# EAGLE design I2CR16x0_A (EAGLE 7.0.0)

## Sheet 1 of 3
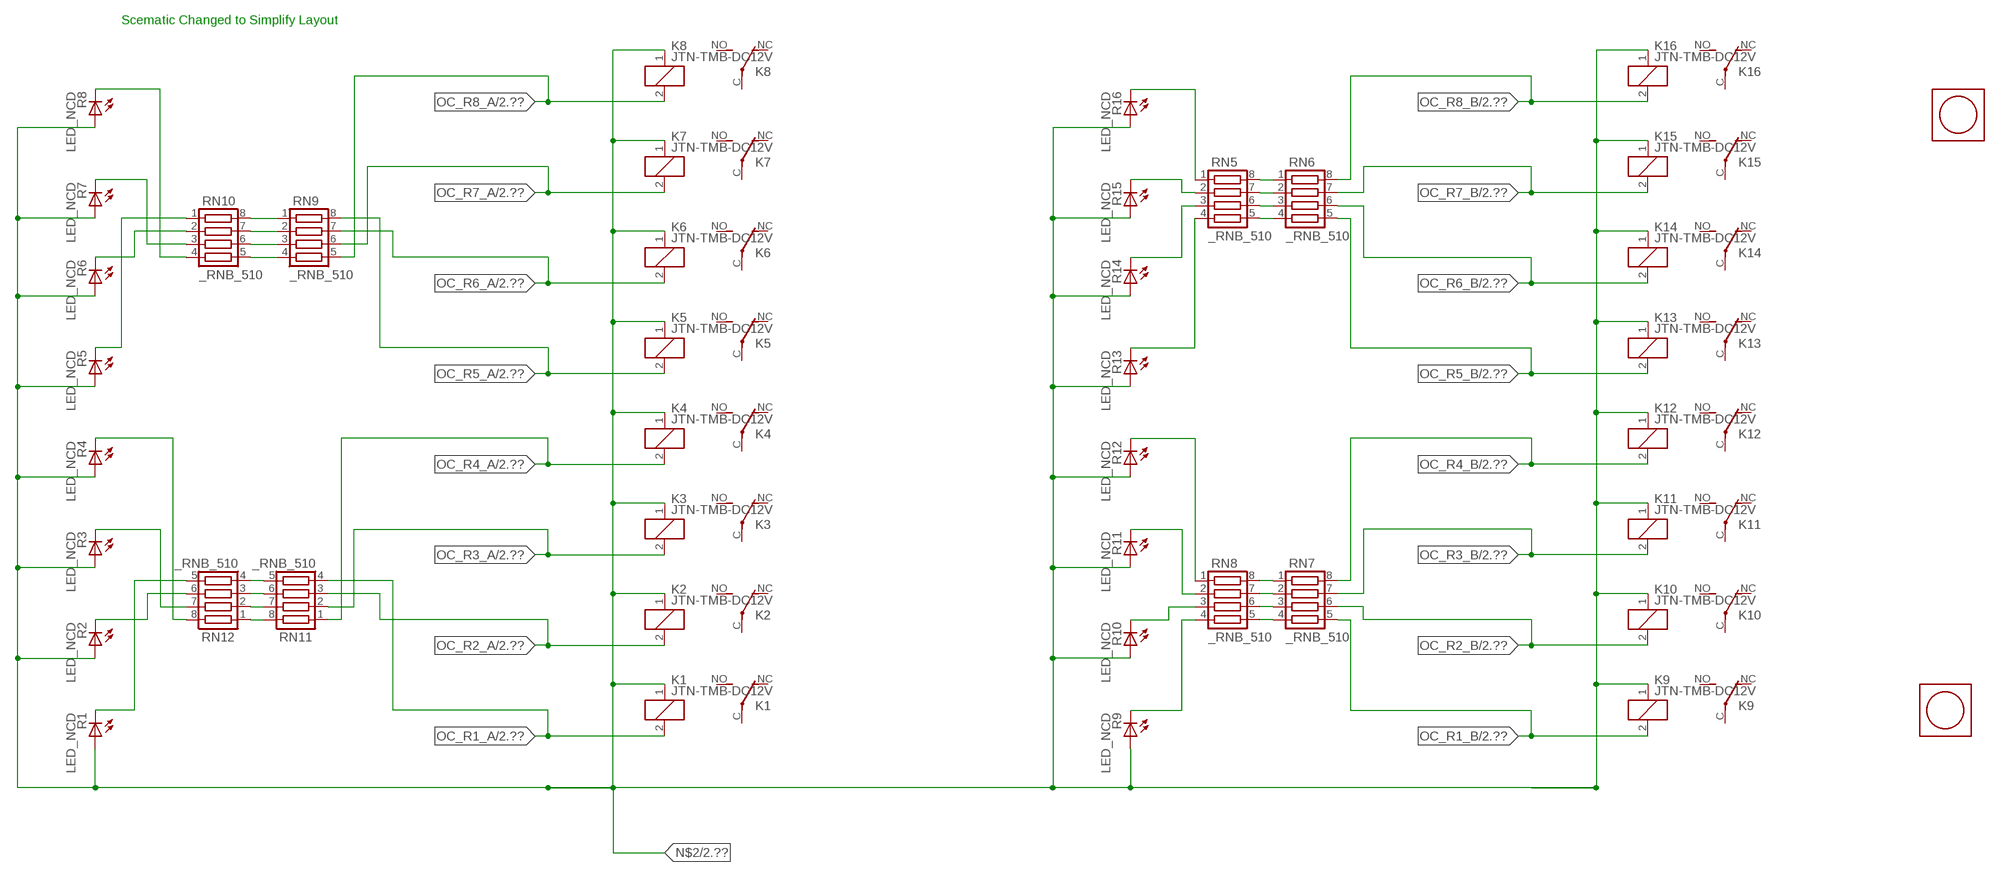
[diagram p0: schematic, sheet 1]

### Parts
K1  JTN-TMB-DC12V  [JT-TMB]
K2  JTN-TMB-DC12V  [JT-TMB]
K3  JTN-TMB-DC12V  [JT-TMB]
K4  JTN-TMB-DC12V  [JT-TMB]
K5  JTN-TMB-DC12V  [JT-TMB]
K6  JTN-TMB-DC12V  [JT-TMB]
K7  JTN-TMB-DC12V  [JT-TMB]
K8  JTN-TMB-DC12V  [JT-TMB]
K9  JTN-TMB-DC12V  [JT-TMB]
K10  JTN-TMB-DC12V  [JT-TMB]
K11  JTN-TMB-DC12V  [JT-TMB]
K12  JTN-TMB-DC12V  [JT-TMB]
K13  JTN-TMB-DC12V  [JT-TMB]
K14  JTN-TMB-DC12V  [JT-TMB]
K15  JTN-TMB-DC12V  [JT-TMB]
K16  JTN-TMB-DC12V  [JT-TMB]
R1  LED_NCD  [CHIPLED_0603]
R2  LED_NCD  [CHIPLED_0603]
R3  LED_NCD  [CHIPLED_0603]
R4  LED_NCD  [CHIPLED_0603]
R5  LED_NCD  [CHIPLED_0603]
R6  LED_NCD  [CHIPLED_0603]
R7  LED_NCD  [CHIPLED_0603]
R8  LED_NCD  [CHIPLED_0603]
R9  LED_NCD  [CHIPLED_0603]
R10  LED_NCD  [CHIPLED_0603]
R11  LED_NCD  [CHIPLED_0603]
R12  LED_NCD  [CHIPLED_0603]
R13  LED_NCD  [CHIPLED_0603]
R14  LED_NCD  [CHIPLED_0603]
R15  LED_NCD  [CHIPLED_0603]
R16  LED_NCD  [CHIPLED_0603]
RN5  _RNB_510  [RNB]
RN6  _RNB_510  [RNB]
RN7  _RNB_510  [RNB]
RN8  _RNB_510  [RNB]
RN9  _RNB_510  [RNB]
RN10  _RNB_510  [RNB]
RN11  _RNB_510  [RNB]
RN12  _RNB_510  [RNB]
U$1  PCB_MOUNTING_HOLE  [PCB_MOUNTING_HOLE]
U$3  PCB_MOUNTING_HOLE  [PCB_MOUNTING_HOLE]

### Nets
N$2: K1.1(C1) K2.1(C1) K3.1(C1) K4.1(C1) K5.1(C1) K6.1(C1) K7.1(C1) K8.1(C1) K9.1(C1) K10.1(C1) K11.1(C1) K12.1(C1) K13.1(C1) K14.1(C1) K15.1(C1) K16.1(C1) R1.A R2.A R3.A R4.A R5.A R6.A R7.A R8.A R9.A R10.A R11.A R12.A R13.A R14.A R15.A R16.A ; also sheet 2,3
N$441: R16.C RN5.1
N$442: RN7.2 RN8.7
N$443: RN7.3 RN8.6
N$444: RN7.4 RN8.5
N$445: R15.C RN5.2
N$447: R13.C RN5.4
N$448: RN5.5 RN6.4
N$449: RN7.1 RN8.8
N$450: R12.C RN8.1
N$451: RN5.6 RN6.3
N$452: R11.C RN8.2
N$453: RN5.7 RN6.2
N$454: RN5.8 RN6.1
N$458: R14.C RN5.3
N$459: R10.C RN8.3
N$463: RN11.5 RN12.4
N$470: R9.C RN8.4
N$473: R1.C RN12.5
N$474: RN11.6 RN12.3
N$475: R2.C RN12.6
N$476: R3.C RN12.7
N$477: RN9.4 RN10.5
N$478: RN9.3 RN10.6
N$479: RN9.2 RN10.7
N$480: RN9.1 RN10.8
N$481: RN11.7 RN12.2
N$482: R5.C RN10.1
N$483: R4.C RN12.8
N$484: R7.C RN10.3
N$485: R8.C RN10.4
N$486: R6.C RN10.2
N$500: RN11.8 RN12.1
OC_R1_A: K1.2(C2) RN11.4 ; also sheet 2
OC_R1_B: K9.2(C2) RN7.5 ; also sheet 2
OC_R2_A: K2.2(C2) RN11.3 ; also sheet 2
OC_R2_B: K10.2(C2) RN7.6 ; also sheet 2
OC_R3_A: K3.2(C2) RN11.2 ; also sheet 2
OC_R3_B: K11.2(C2) RN7.7 ; also sheet 2
OC_R4_A: K4.2(C2) RN11.1 ; also sheet 2
OC_R4_B: K12.2(C2) RN7.8 ; also sheet 2
OC_R5_A: K5.2(C2) RN9.8 ; also sheet 2
OC_R5_B: K13.2(C2) RN6.5 ; also sheet 2
OC_R6_A: K6.2(C2) RN9.7 ; also sheet 2
OC_R6_B: K14.2(C2) RN6.6 ; also sheet 2
OC_R7_A: K7.2(C2) RN9.6 ; also sheet 2
OC_R7_B: K15.2(C2) RN6.7 ; also sheet 2
OC_R8_A: K8.2(C2) RN9.5 ; also sheet 2
OC_R8_B: K16.2(C2) RN6.8 ; also sheet 2
Unconnected: K1.C(COM) K1.NC K1.NO K2.C(COM) K2.NC K2.NO K3.C(COM) K3.NC K3.NO K4.C(COM) K4.NC K4.NO K5.C(COM) K5.NC K5.NO K6.C(COM) K6.NC K6.NO K7.C(COM) K7.NC K7.NO K8.C(COM) K8.NC K8.NO K9.C(COM) K9.NC K9.NO K10.C(COM) K10.NC K10.NO K11.C(COM) K11.NC K11.NO K12.C(COM) K12.NC K12.NO K13.C(COM) K13.NC K13.NO K14.C(COM) K14.NC K14.NO K15.C(COM) K15.NC K15.NO K16.C(COM) K16.NC K16.NO

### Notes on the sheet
- Scematic Changed to Simplify Layout

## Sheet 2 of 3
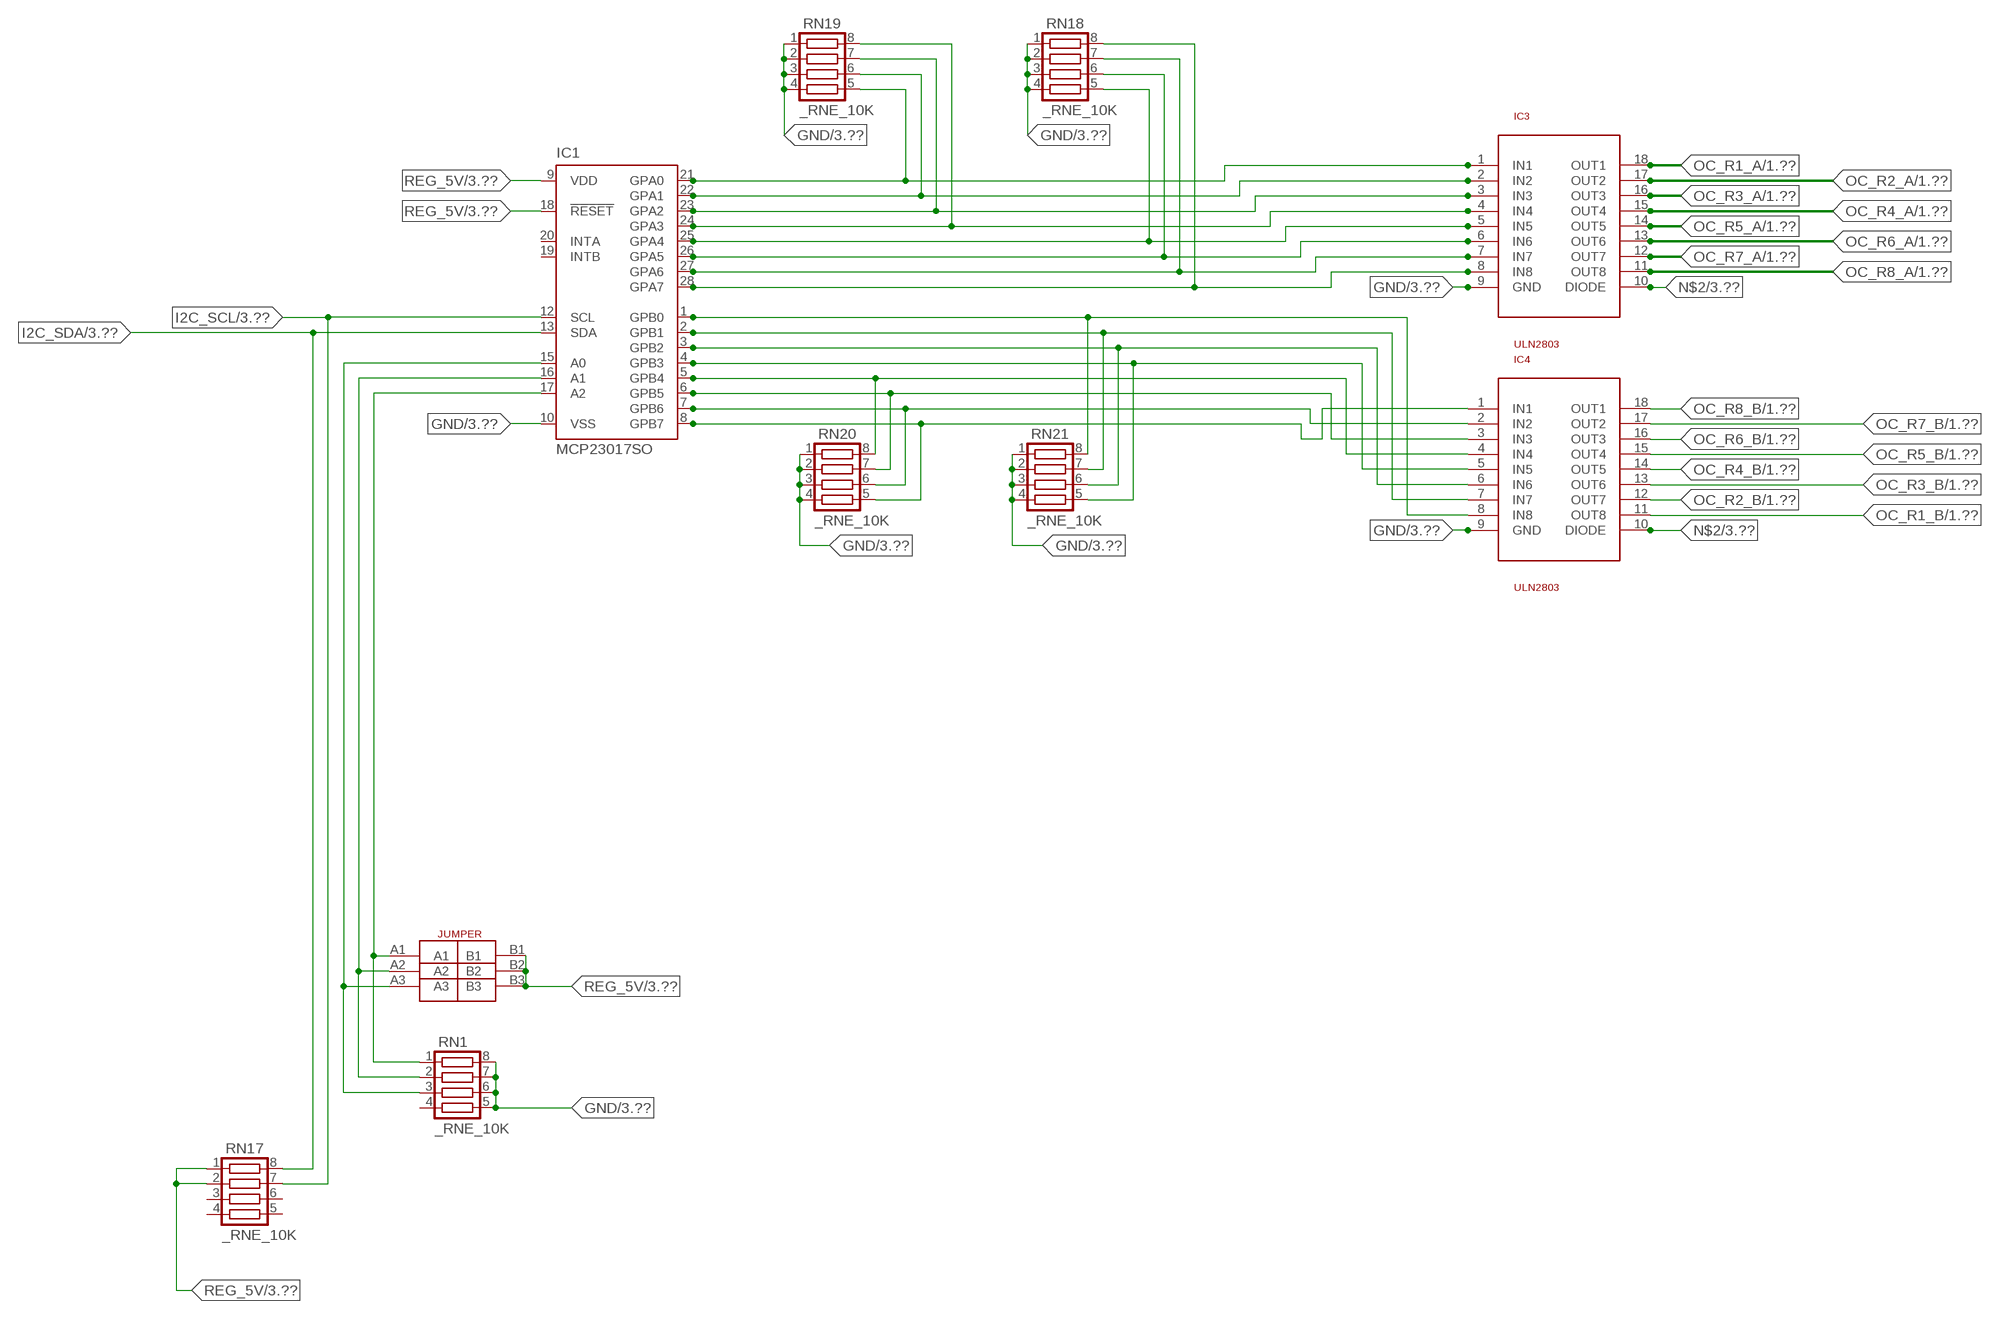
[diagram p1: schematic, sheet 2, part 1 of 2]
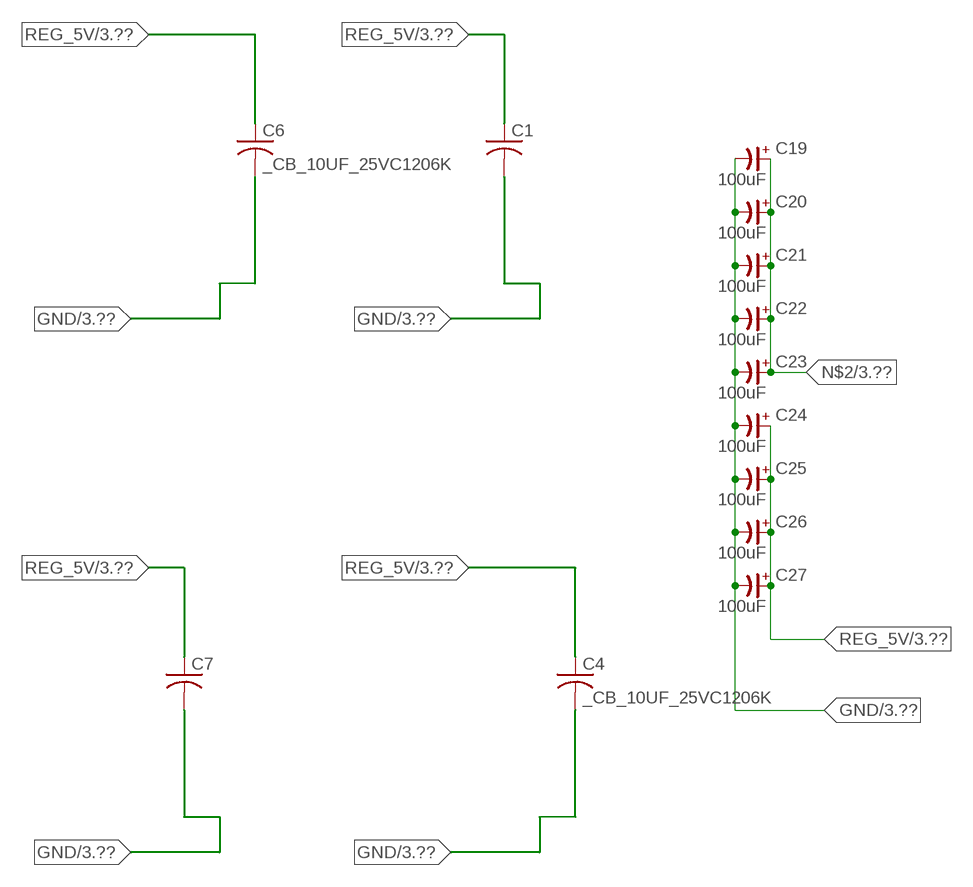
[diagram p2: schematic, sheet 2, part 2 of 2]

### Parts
C1  _CA_.10UF_50VC1206K  [_CA_.1UF_50V]
C4  _CB_10UF_25VC1206K  [_CB_10UF_25V]
C6  _CB_10UF_25VC1206K  [_CB_10UF_25V]
C7  _CA_.10UF_50VC1206K  [_CA_.1UF_50V]
C19  100uF  CP-E-025X060  [E-025X060]
C20  100uF  CP-E-025X060  [E-025X060]
C21  100uF  CP-E-025X060  [E-025X060]
C22  100uF  CP-E-025X060  [E-025X060]
C23  100uF  CP-E-025X060  [E-025X060]
C24  100uF  CP-E-025X060  [E-025X060]
C25  100uF  CP-E-025X060  [E-025X060]
C26  100uF  CP-E-025X060  [E-025X060]
C27  100uF  CP-E-025X060  [E-025X060]
IC1  MCP23017SO  [SO28W]
IC3  ULN2803  [SO18L]
IC4  ULN2803  [SO18L]
JP1  JUMPER_3X2  [JUMPER_3X2]
RN1  _RNE_10K  [RNE]
RN17  _RNE_10K  [RNE]
RN18  _RNE_10K  [RNE]
RN19  _RNE_10K  [RNE]
RN20  _RNE_10K  [RNE]
RN21  _RNE_10K  [RNE]

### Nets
GND: C1.2 C4.2 C6.2 C7.2 C19.- C20.- C21.- C22.- C23.- C24.- C25.- C26.- C27.- IC1.10(VSS) IC3.9(GND) IC4.9(GND) RN1.5 RN1.6 RN1.7 RN1.8 RN18.1 RN18.2 RN18.3 RN18.4 RN19.1 RN19.2 RN19.3 RN19.4 RN20.1 RN20.2 RN20.3 RN20.4 RN21.1 RN21.2 RN21.3 RN21.4 ; also sheet 3
I2C_SCL: IC1.12(SCL) RN17.7 ; also sheet 3
I2C_SDA: IC1.13(SDA) RN17.8 ; also sheet 3
N$2: C19.+ C20.+ C21.+ C22.+ C23.+ IC3.10(DIODE) IC4.10(DIODE) ; also sheet 1,3
N$4: IC1.15(A0) JP1.A3 RN1.3
N$405: IC1.21(GPA0) IC3.1(IN1) RN19.5
N$406: IC1.25(GPA4) IC3.5(IN5) RN18.5
N$407: IC1.26(GPA5) IC3.6(IN6) RN18.6
N$408: IC1.16(A1) JP1.A2 RN1.2
N$409: IC1.22(GPA1) IC3.2(IN2) RN19.6
N$410: IC1.23(GPA2) IC3.3(IN3) RN19.7
N$411: IC1.24(GPA3) IC3.4(IN4) RN19.8
N$416: IC1.1(GPB0) IC4.8(IN8) RN21.8
N$417: IC1.2(GPB1) IC4.7(IN7) RN21.7
N$418: IC1.3(GPB2) IC4.6(IN6) RN21.6
N$419: IC1.4(GPB3) IC4.5(IN5) RN21.5
N$420: IC1.5(GPB4) IC4.4(IN4) RN20.8
N$421: IC1.6(GPB5) IC4.3(IN3) RN20.7
N$422: IC1.7(GPB6) IC4.2(IN2) RN20.6
N$423: IC1.8(GPB7) IC4.1(IN1) RN20.5
N$498: IC1.17(A2) JP1.A1 RN1.1
N$525: IC1.27(GPA6) IC3.7(IN7) RN18.7
N$526: IC1.28(GPA7) IC3.8(IN8) RN18.8
OC_R1_A: IC3.18(OUT1) ; also sheet 1
OC_R1_B: IC4.11(OUT8) ; also sheet 1
OC_R2_A: IC3.17(OUT2) ; also sheet 1
OC_R2_B: IC4.12(OUT7) ; also sheet 1
OC_R3_A: IC3.16(OUT3) ; also sheet 1
OC_R3_B: IC4.13(OUT6) ; also sheet 1
OC_R4_A: IC3.15(OUT4) ; also sheet 1
OC_R4_B: IC4.14(OUT5) ; also sheet 1
OC_R5_A: IC3.14(OUT5) ; also sheet 1
OC_R5_B: IC4.15(OUT4) ; also sheet 1
OC_R6_A: IC3.13(OUT6) ; also sheet 1
OC_R6_B: IC4.16(OUT3) ; also sheet 1
OC_R7_A: IC3.12(OUT7) ; also sheet 1
OC_R7_B: IC4.17(OUT2) ; also sheet 1
OC_R8_A: IC3.11(OUT8) ; also sheet 1
OC_R8_B: IC4.18(OUT1) ; also sheet 1
REG_5V: C1.1 C4.1 C6.1 C7.1 C24.+ C25.+ C26.+ C27.+ IC1.9(VDD) IC1.18(!RESET) JP1.B1 JP1.B2 JP1.B3 RN17.1 RN17.2 ; also sheet 3
Unconnected: IC1.19(INTB) IC1.20(INTA) RN1.4 RN17.3 RN17.4 RN17.5 RN17.6

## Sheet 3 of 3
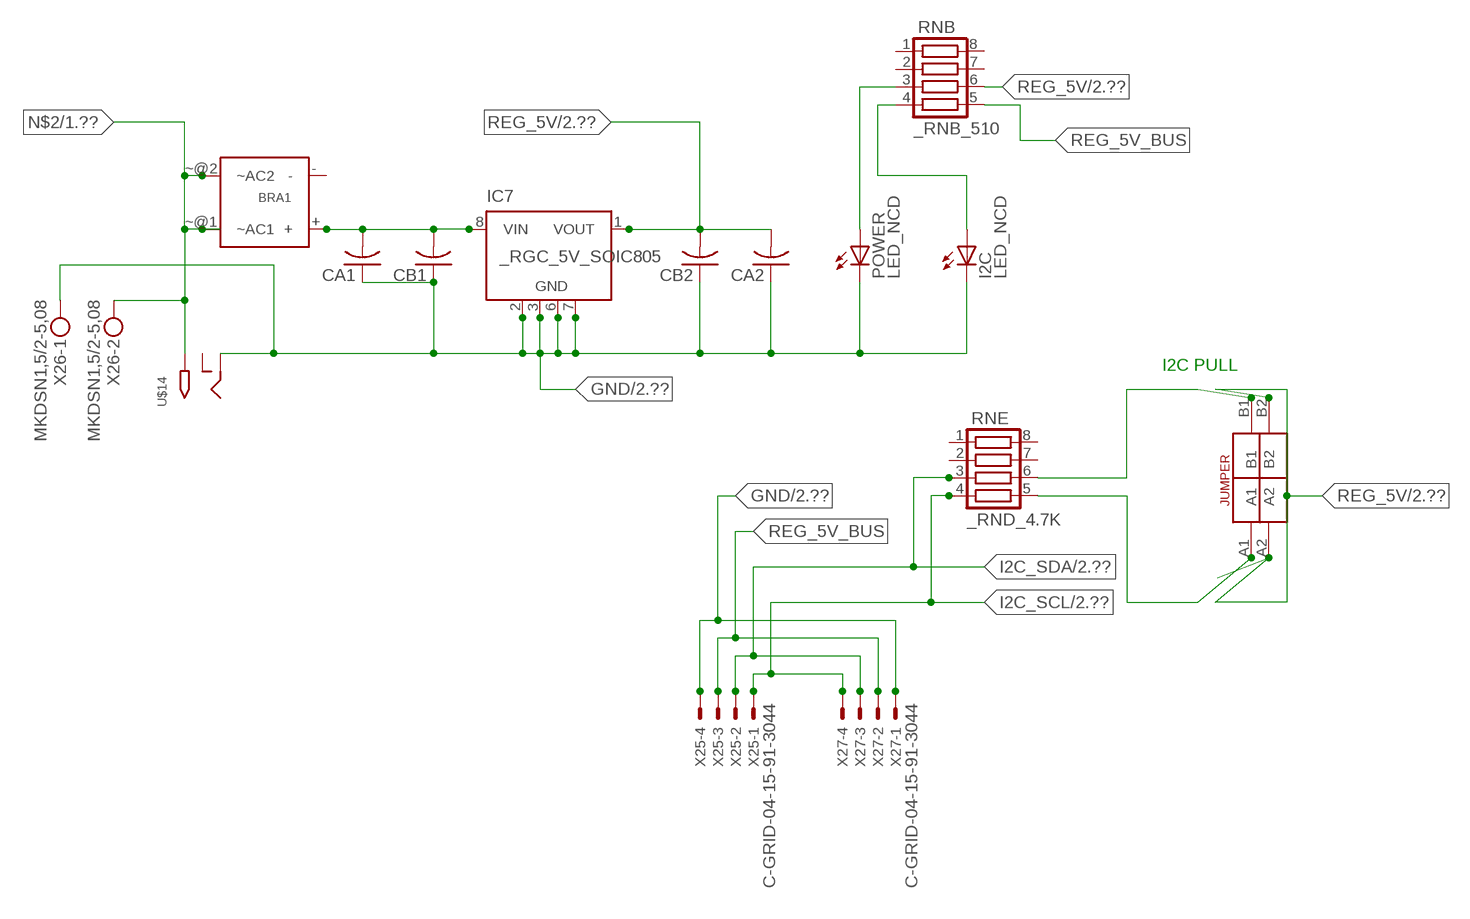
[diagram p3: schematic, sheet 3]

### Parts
BRA1  MB2S_  [MB2S]
CA1  CC1206KRX7R9BB104C1206K  [CC1206KRX7R9BB104]
CA2  CC1206KRX7R9BB104C1206K  [CC1206KRX7R9BB104]
CB1  TMK316F106ZL-TC1206K  [TMK316F106ZL-T]
CB2  TMK316F106ZL-TC1206K  [TMK316F106ZL-T]
I2C  LED_NCD  [CHIPLED_0603]
IC7  _RGC_5V_SOIC805  [_RGC_5V_SOIC8]
POWER  LED_NCD  [CHIPLED_0603]
RNB  _RNB_510  [RNB]
RNE  _RND_4.7K  [RND]
U$14  2.1MMJACK  [PJ-102A]
U$16  JUMPER_2X2  [JUMPER_2X2]
X25  C-GRID-04-15-91-3044  [15-91-04]
X26  MKDSN1,5/2-5,08  [MKDSN1,5/2-5,08]
X27  C-GRID-04-15-91-3044  [15-91-04]

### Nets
GND: CA1.1 CA2.1 CB1.1 CB2.1 I2C.C IC7.2(GND) IC7.3(GND) IC7.6(GND) IC7.7(GND) POWER.C U$14.RING X25.4 X26.1 X27.1 ; also sheet 2
I2C_SCL: RNE.4 X25.1 X27.4 ; also sheet 2
I2C_SDA: RNE.3 X25.2 X27.3 ; also sheet 2
N$2: BRA1.~@1(~AC1) BRA1.~@2(~AC2) U$14.TIP X26.2 ; also sheet 1,2
N$513: BRA1.+ CA1.2 CB1.2 IC7.8(VIN)
N$515: POWER.A RNB.3
N$516: I2C.A RNB.4
N$517: RNE.5 U$16.A1
N$518: RNE.6 U$16.B1
REG_5V: CA2.2 CB2.2 IC7.1(VOUT) RNB.6 U$16.A2 U$16.B2 ; also sheet 2
REG_5V_BUS: RNB.5 X25.3 X27.2
Unconnected: BRA1.- IC7.4(NC) IC7.5(NC) RNB.1 RNB.2 RNB.7 RNB.8 RNE.1 RNE.2 RNE.7 RNE.8 U$14.RING_SW

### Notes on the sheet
- I2C PULL

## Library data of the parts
BRA1 = NCD_ULTIMATE_LIBRARY:MB2S: Bridge Rectifier BRA MB2S 200V 500ma Digikey MB2S-TPMSTR-ND/MB2S-TP
C1 C7 = NCD_ULTIMATE_LIBRARY:_CA_.10UF_50V: Capacitor .1uF SMT
C4 C6 = NCD_ULTIMATE_LIBRARY:_CB_10UF_25V: Capacitor 10uF SMT
C19-C27 = NCD_ULTIMATE_LIBRARY:CP-: Capacitors All Kinds POLARIZED CAP
CA1 CA2 = NCD_ULTIMATE_LIBRARY:CC1206KRX7R9BB104: Capacitor CA .1uF 50V SMT C1206K CC1206KRX7R9BB104
CB1 CB2 = NCD_ULTIMATE_LIBRARY:TMK316F106ZL-T: Capacitor CB 10uF SMT 1206 TMK316F106ZL-T
I2C POWER R1-R16 = NCD_ULTIMATE_bhaskar:LED_NCD
IC1 = NCD_ULTIMATE_LIBRARY:MCP23017: Semiconductor Port Expander I/O 16-Bit I2C http://ww1.microchip.com/downloads/en/DeviceDoc/21952a.pdf Source: http://ww1.microchip.com/downloads/en/DeviceDoc/21952a.pdf
IC3 IC4 = NCD_ULTIMATE_LIBRARY:ULN2803: Semiconductor 8 O.C. N-Channel Transistor Driver Digikey ULN2803AFWGCELTR-ND/ULN2803AFWG,C,EL
IC7 = NCD_ULTIMATE_LIBRARY:_RGC_5V_SOIC8: Regulator Linear 5V Chip Positive VOLTAGE REGULATOR Digikey 497-7267-2-ND/L78L05CD13TR
JP1 = NCD_ULTIMATE_CONNECTORS:JUMPER_3X2
K1-K16 = NCD_ULTIMATE_LIBRARY:JT?-*: RELAY COMPACT ECONOMICAL 30 AMP. RELAY NAiS Source: http://www.mew-europe.com/.. en_ds_61212_0000.pdf
RN1 RN17-RN21 = NCD_ULTIMATE_LIBRARY:_RNE_10K: Resistor Array RNE SMT 10K x 4 Single Resistor Source: http://www.ctscorp.com/components/Datasheets/CTSChipArrayDs.pdf Digikey 742C083103JPTR-ND/742C083103JP; OC_FARNELL: unknown; OC_NEWARK: unknown
RN5-RN12 RNB = NCD_ULTIMATE_LIBRARY:_RNB_510: Resistor Array RNB SMT 510 x 4 Single Resistor Source: http://www.ctscorp.com/components/Datasheets/CTSChipArrayDs.pdf Digikey 742C083511JPTR-ND/ 742C083511JP; OC_FARNELL: unknown; OC_NEWARK: unknown
RNE = NCD_ULTIMATE_LIBRARY:_RND_4.7K: Resistor Array RND SMT 4.7K x 4 Single Resistor Source: http://www.ctscorp.com/components/Datasheets/CTSChipArrayDs.pdf Digikey 742C083472JPTR-ND/742C083472JP; OC_FARNELL: unknown; OC_NEWARK: unknown
U$1 U$3 = NCD_ULTIMATE_CONNECTORS:PCB_MOUNTING_HOLE
U$14 = NCD_ULTIMATE_CONNECTORS:2.1MMJACK: 2.1mm x 5.5mm DC jack with internal switch. Digikey part #PJ-102A, 4UCON part #05537 By microbuilder.eu
U$16 = NCD_ULTIMATE_CONNECTORS:JUMPER_2X2
X25 X27 = NCD_ULTIMATE_CONNECTORS:C-GRID-04: CONNECTOR 4-Pos I2C wire to board 2.54 mm (0.100") pitch header Digikey WM1342-ND/0015912045; OC_FARNELL: unknown; OC_NEWARK: unknown
X26 = NCD_ULTIMATE_CONNECTORS:MKDSN1,5/2-5,08: MKDSN 1,5/ 2-5,08 Printklemme

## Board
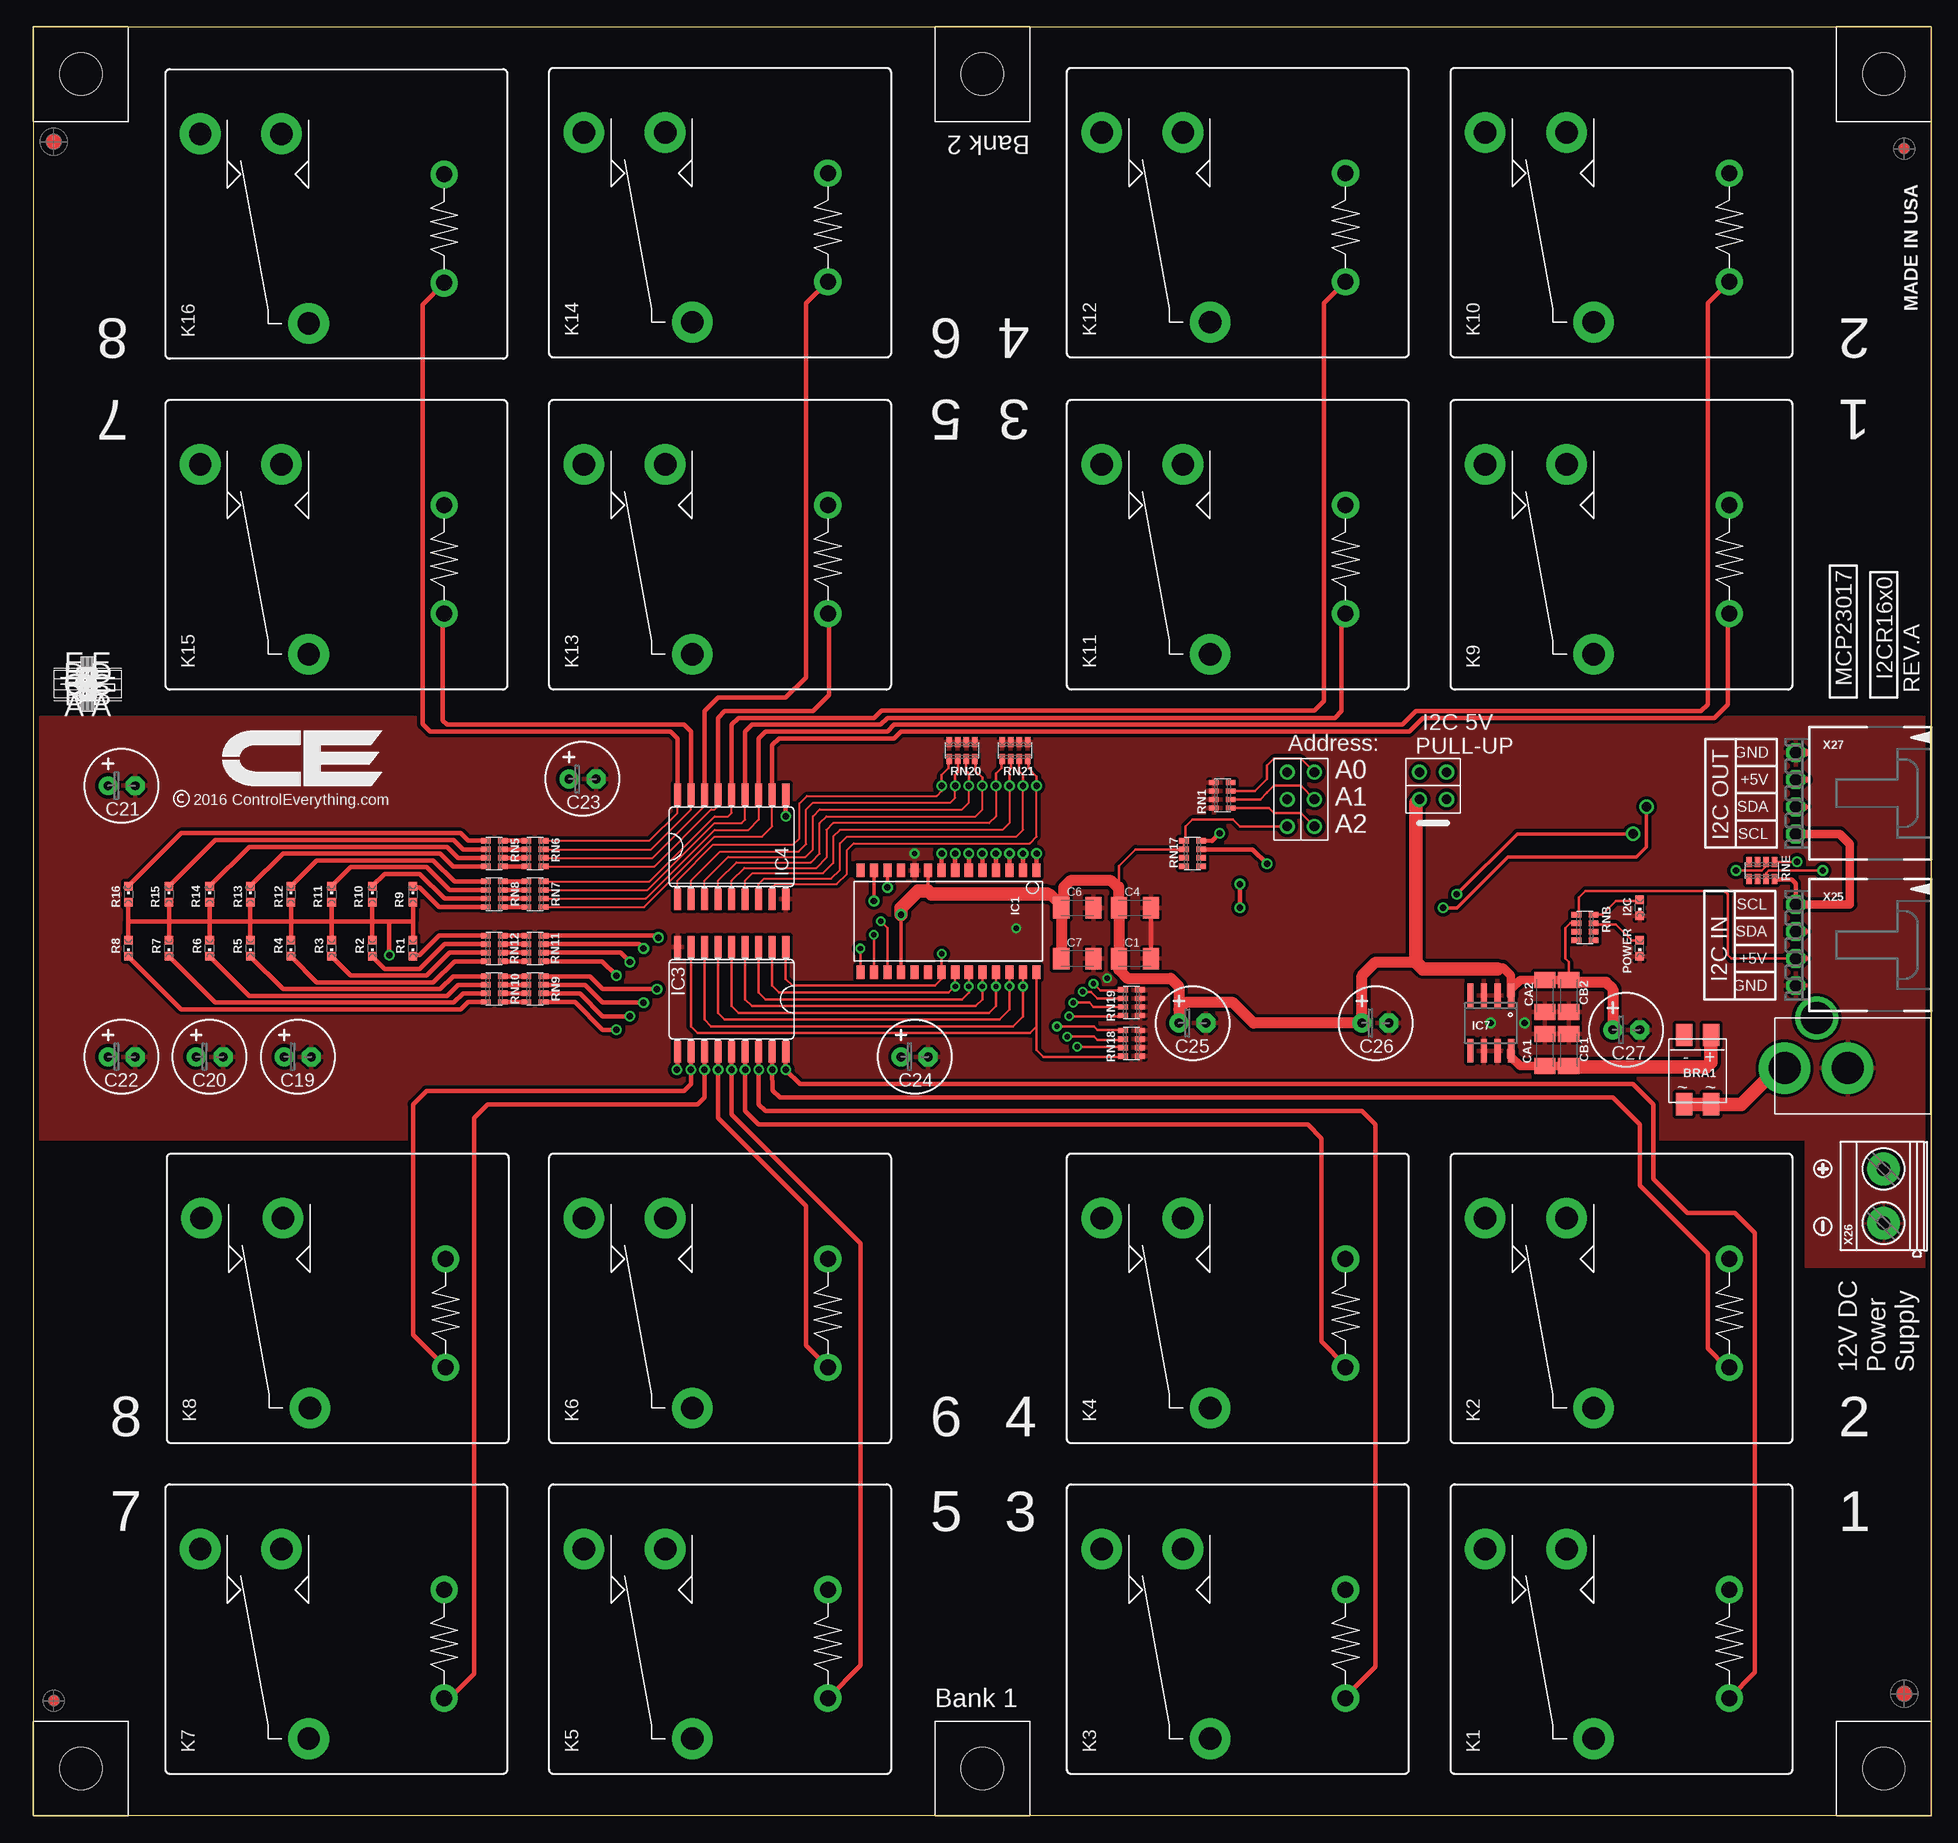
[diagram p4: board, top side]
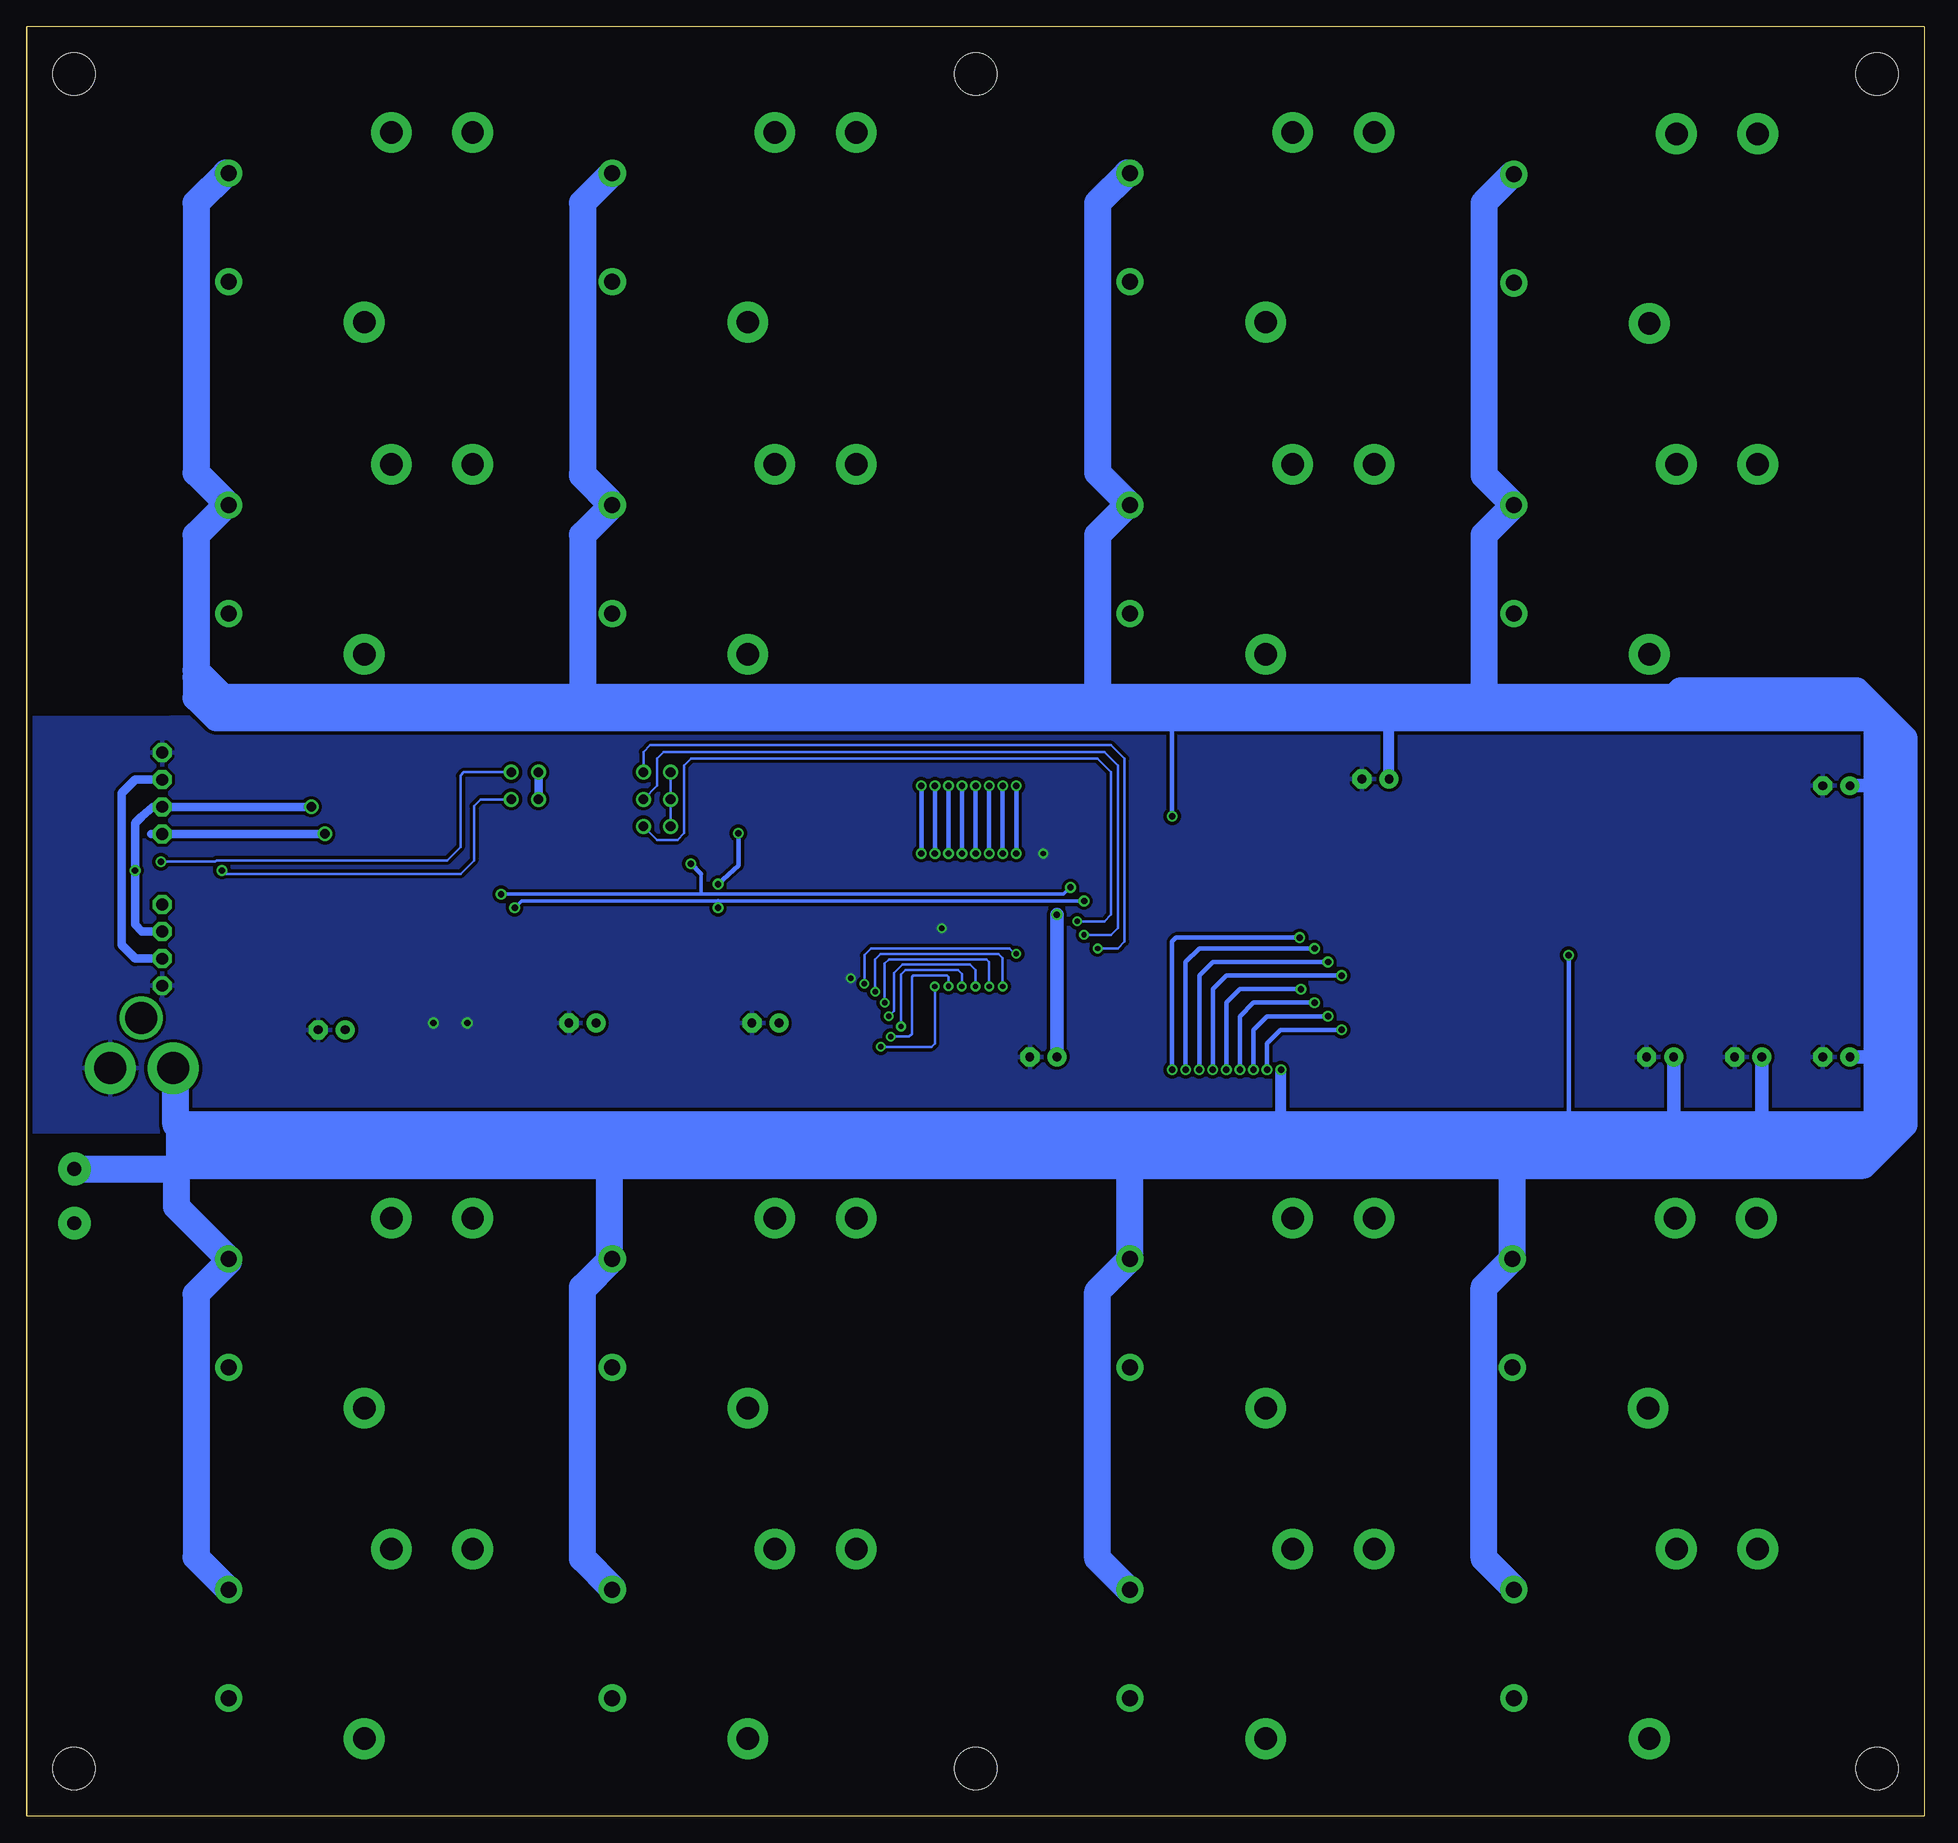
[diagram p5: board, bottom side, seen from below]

Size 177.8 x 167.65 mm. Coordinates in mm from the lower left corner, seen from the top.
Outline: 177.78,0 177.78,167.65 0,167.65 0,0.01 177.8,0.01 177.8,167.65
Copper layers (1*16): Top 0.035mm / dielectric 1.5mm / Bottom 0.035mm
Design rules "default *": minimum track width 6mil, minimum drill 12mil, track to track 5mil, track to pad 5mil, pad to pad 5mil, via to via 5mil, smd to smd 5mil, copper to edge 20mil, drill to drill 8mil, minimum pad ring 10mil, minimum via ring 8mil, stop-mask expansion 4mil, vias tented up to drill 0mil, thermal gap 10mil

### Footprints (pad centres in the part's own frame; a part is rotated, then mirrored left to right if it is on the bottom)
MB2S = smd 1.55 x 2.1: + 0,-6.5; - 2.54,-6.5; ~@1 0,0; ~@2 2.54,0
_CA_.1UF_50V = smd 1.5 x 2: 1 -1.5,0; 2 1.5,0
_CB_10UF_25V = smd 1.5 x 2: 1 -1.5,0; 2 1.5,0
E-025X060 = drill 0.813 pad 1.778: + -1.27,0 | drill 0.813 pad 1.778 octagon: - 1.27,0
CC1206KRX7R9BB104 = smd 1.5 x 2: 1 -1.5,0; 2 1.5,0
TMK316F106ZL-T = smd 1.5 x 2: 1 -1.5,0; 2 1.5,0
CHIPLED_0603 = smd 0.8 x 0.8: A 0,-0.75; C 0,0.75
SO28W = smd 0.762 x 1.27: 1 -7.62,-4.78; 2 -6.35,-4.78; 3 -5.08,-4.78; 4 -3.81,-4.78; 5 -2.54,-4.78; 6 -1.27,-4.78; 7 0,-4.78; 8 1.27,-4.78; 9 2.54,-4.78; 10 3.81,-4.78; 11 5.08,-4.78; 12 6.35,-4.78; 13 7.62,-4.78; 14 8.89,-4.78; 15 8.89,4.78; 16 7.62,4.78; 17 6.35,4.78; 18 5.08,4.78; 19 3.81,4.78; 20 2.54,4.78; 21 1.27,4.78; 22 0,4.78; 23 -1.27,4.78; 24 -2.54,4.78; 25 -3.81,4.78; 26 -5.08,4.78; 27 -6.35,4.78; 28 -7.62,4.78
SO18L = smd 0.66 x 2.032: 1 -5.08,-4.902; 2 -3.81,-4.902; 3 -2.54,-4.902; 4 -1.27,-4.902; 5 0,-4.902; 6 1.27,-4.902; 7 2.54,-4.902; 8 3.81,-4.902; 9 5.08,-4.902; 10 5.08,4.902; 11 3.81,4.902; 12 2.54,4.902; 13 1.27,4.902; 14 0,4.902; 15 -1.27,4.902; 16 -2.54,4.902; 17 -3.81,4.902; 18 -5.08,4.902
_RGC_5V_SOIC8 = smd 0.6 x 2.2: 1 -1.905,-2.6; 2 -0.635,-2.6; 3 0.635,-2.6; 4 1.905,-2.6; 5 1.905,2.6; 6 0.635,2.6; 7 -0.635,2.6; 8 -1.905,2.6
JUMPER_3X2 = drill 0.9: A1 0,5.08; A2 0,2.54; A3 0,0; B1 2.54,5.08; B2 2.54,2.54; B3 2.54,0
JT-TMB = drill 1.5 pad 2.54: 1 5.08,0; 2 -5.08,0 | drill 2.1 pad 3.81: C -8.89,12.7; NC 8.89,22.86; NO 8.89,15.24
RNE = smd 0.5 x 0.9: 1 -1.2,-0.8; 2 -0.4,-0.8; 3 0.4,-0.8; 4 1.2,-0.8; 5 1.2,0.8; 6 0.4,0.8; 7 -0.4,0.8; 8 -1.2,0.8
RNB = smd 0.5 x 0.9: 1 -1.2,-0.8; 2 -0.4,-0.8; 3 0.4,-0.8; 4 1.2,-0.8; 5 1.2,0.8; 6 0.4,0.8; 7 -0.4,0.8; 8 -1.2,0.8
RND = smd 0.5 x 0.9: 1 -1.2,-0.8; 2 -0.4,-0.8; 3 0.4,-0.8; 4 1.2,-0.8; 5 1.2,0.8; 6 0.4,0.8; 7 -0.4,0.8; 8 -1.2,0.8
PCB_MOUNTING_HOLE = hole 3.962: 4.445,4.445
PJ-102A = drill 3 pad 4.8: RING 0.1,-3.39; TIP 0.1,-9.29 | drill 3 pad 3.251: RING_SW -4.6,-6.29
JUMPER_2X2 = drill 0.9: A1 0,2.54; A2 0,0; B1 2.54,2.54; B2 2.54,0
15-91-04 = drill 1.1 pad 1.778 octagon: 1 -3.81,-7.62; 2 -1.27,-7.62; 3 1.27,-7.62; 4 3.81,-7.62
MKDSN1,5/2-5,08 = drill 1.3 pad 3.048: 1 -2.561,0.025; 2 2.519,0.025

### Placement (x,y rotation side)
BRA1  157.16,66.69 180 top
C1  103.19,80.34 0 top
C4  103.19,85.1 0 top
C6  97.79,85.1 0 top
C7  97.79,80.34 0 top
C19  24.77,71.13 0 top
C20  16.51,71.13 0 top
C21  8.26,96.53 0 top
C22  8.26,71.13 0 top
C23  51.44,97.17 0 top
C24  82.55,71.13 0 top
C25  108.58,74.31 0 top
C26  125.73,74.31 0 top
C27  149.22,73.67 0 top
CA1  141.6,71.77 270 top
CA2  141.6,76.85 90 top
CB1  143.83,71.77 270 top
CB2  143.83,76.85 90 top
I2C  150.5,85.1 180 top
IC1  86.36,83.83 180 top
IC3  65.41,76.53 180 top
IC4  65.41,90.82 0 top
IC7  136.53,74.31 180 top
JP1  120.02,97.8 180 top
K1  158.88,16.14 90 top
K2  158.88,47.13 90 top
K3  122.94,16.14 90 top
K4  122.94,47.13 90 top
K5  74.42,16.14 90 top
K6  74.42,47.13 90 top
K7  38.48,16.14 90 top
K8  38.61,47.13 90 top
K9  158.88,117.74 90 top
K10  158.88,148.86 90 top
K11  122.94,117.74 90 top
K12  122.94,148.86 90 top
K13  74.42,117.74 90 top
K14  74.42,148.86 90 top
K15  38.48,117.74 90 top
K16  38.48,148.73 90 top
POWER  150.5,81.29 180 top
R1  35.56,81.29 180 top
R2  31.75,81.29 180 top
R3  27.94,81.29 180 top
R4  24.13,81.29 180 top
R5  20.32,81.29 180 top
R6  16.51,81.29 180 top
R7  12.7,81.29 180 top
R8  8.89,81.29 180 top
R9  35.56,86.37 0 top
R10  31.75,86.37 0 top
R11  27.94,86.37 0 top
R12  24.13,86.37 0 top
R13  20.32,86.37 0 top
R14  16.51,86.37 0 top
R15  12.7,86.37 0 top
R16  8.89,86.37 0 top
RN1  111.38,95.64 90 top
RN5  43.18,90.18 270 top
RN6  46.99,90.18 270 top
RN7  46.99,86.37 270 top
RN8  43.18,86.37 270 top
RN9  46.99,77.48 270 top
RN10  43.18,77.48 270 top
RN11  46.99,81.29 90 top
RN12  43.18,81.29 90 top
RN17  108.58,90.18 270 top
RN18  102.87,72.4 90 top
RN19  102.87,76.21 90 top
RN20  87,99.83 180 top
RN21  91.95,99.83 180 top
RNB  145.35,83.26 90 top
RNE  161.93,88.59 0 top
U$1  93.34,158.76 90 top
U$3  177.8,158.76 90 top
U$5  PCB_MOUNTING_HOLE  [PCB_MOUNTING_HOLE]  0,8.9 270 top
U$9  PCB_MOUNTING_HOLE  [PCB_MOUNTING_HOLE]  8.89,158.76 90 top
U$10  PCB_MOUNTING_HOLE  [PCB_MOUNTING_HOLE]  84.45,8.9 270 top
U$11  PCB_MOUNTING_HOLE  [PCB_MOUNTING_HOLE]  168.91,8.9 270 top
U$12  PCB_MOUNTING_HOLE  [PCB_MOUNTING_HOLE]  0,8.9 270 top
U$14  173.35,70.18 270 top
U$15  [VISION_REF15]  175.26,11.44 90 top
U$16  129.86,97.8 270 top
U$18  [VISION_REF10]  175.26,156.22 90 top
U$21  [ICON_USA]  176.53,140.98 90 top
U$22  [ICON_MINUS]  167.64,55.26 90 top
U$23  [VISION_REF15]  1.91,156.86 90 top
U$24  [ICON_PLUS]  167.64,60.66 0 top
U$28  [VISION_REF10]  1.91,10.81 90 top
X25  172.72,81.61 270 top
X26  173.35,58.12 90 top
X27  172.72,95.83 270 top

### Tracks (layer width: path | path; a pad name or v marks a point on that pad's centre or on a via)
GND  (via drill 0.5, 0.6)
  Top 0.406: C1.2 C4.2 | 165.99,77.8 X25.4
  Top 0.813: X27.1 165.99,99.64
  other vias: 139.7,74.31 136.53,74.31 100.58,78.5 82.55,90.18 92.08,83.2
  pour Top (isolate 0.305): -5.71,63.51 -5.71,102.88 177.48,102.88 177.48,63.51
  pour Top (isolate 0.305): 177.48,51.45 166.05,51.45 166.05,63.51 177.48,63.51
  pour Bottom (isolate 0.305): -3.17,103.52 177.16,102.88 177.16,64.15 -3.17,64.15
I2C_SCL  (via drill 0.6, 0.9)
  Top 0.305: v80.01,87.01 IC1.12 | v149.86,92.02 139,92.02 v133.35,86.37
  Top 0.406: RN17.7 114.22,90.58 v115.57,89.23 | X25.1 165.1,87.39 164.72,87.77 163.15,87.77 RNE.4
  Top 0.813: X25.1 170.18,85.42 170.18,91.08 169.24,92.02 X27.4
  Bottom 0.305: v133.35,86.37 114.62,86.37 | 114.62,86.37 80.64,86.37 v80.01,87.01 | 114.62,88.28 114.62,86.37
  Bottom 0.406: v115.57,89.23 114.62,88.28
  Bottom 0.813: v149.86,92.02 X27.4 166.12,92.02
I2C_SDA  (via drill 0.6, 0.9)
  Top 0.254: RNE.3 162.32,88.36 162.56,88.59 v167.64,88.59
  Top 0.305: v78.74,85.74 IC1.13 | v151.13,94.56 151.13,90.82 150.18,89.87 138.11,89.87 133.35,85.1 v132.08,85.1
  Top 0.406: RN17.8 110.4,91.36 v111.12,92.09 | v113.03,87.32 v113.03,85.1
  Top 0.61: X27.3 165.99,94.56 | X25.2 165.99,82.88
  Bottom 0.305: v78.74,85.74 113.03,85.74 131.44,85.74 v132.08,85.1
  Bottom 0.406: v111.12,92.09 111.12,89.04 v113.03,87.32 | v113.03,85.1 113.03,85.74 | 165.99,82.88 X25.2
  Bottom 0.813: 165.99,82.88 167,82.88 167.64,83.51 v167.64,88.59 167.64,93.04 167,93.67 165.99,94.56 X27.3 v151.13,94.56
N$2  (via drill 0.6)
  Top 0.305: 35.56,83.83 R1.A
  Top 0.406: IC4.10 v70.48,93.67 | R8.A 8.89,83.83 | R15.A 12.7,83.83 | R6.A 16.51,83.83 | 20.32,83.83 R13.A | R4.A 24.13,83.83 | R3.A 27.94,83.83 | R2.A 31.75,83.83 | R16.A 8.89,83.83 | 8.89,83.83 12.7,83.83 | R7.A 12.7,83.83 | 12.7,83.83 16.51,83.83 | R14.A 16.51,83.83 | 16.51,83.83 20.32,83.83 | R5.A 20.32,83.83 | 20.32,83.83 24.13,83.83 | R12.A 24.13,83.83 | 24.13,83.83 27.94,83.83 | R11.A 27.94,83.83 | 27.94,83.83 31.75,83.83 | R10.A 31.75,83.83 | R9.A 35.56,83.83 | 35.56,81.93 35.56,83.83 | 35.56,83.83 33.34,83.83 | 31.75,83.83 33.34,83.83 | 33.34,83.83 v33.34,80.66 | IC3.10 60.33,70.5 v60.29,69.93
  Top 1.27: U$14.TIP 163.41,70.08 160.02,66.69 BRA1.~@1 BRA1.~@2
  Bottom 0.406: v70.48,93.67 70.48,102.25 69.85,102.88 | v33.34,80.66 33.34,64.78 | 60.39,65.1 60.71,64.78
  Bottom 1.016: 60.39,65.1 60.29,65.1 v60.29,69.93 | 51.44,102.25 50.8,102.88 | 2.54,65.42 1.91,64.78 | C23.+ 50.16,102.88
  Bottom 1.27: C22.+ 4.45,71.13 | C21.+ 4.45,96.53 | C19.+ 23.5,64.78 | C20.+ 15.24,64.78
  Bottom 2.54: 2.54,66.05 2.54,66.69 | 2.54,100.34 2.54,66.69 | 2.54,66.69 3.17,66.05 1.91,64.78 | 1.91,64.78 1.91,100.98 6.35,105.42 22.86,105.42 23.5,104.79 | 163.83,64.78 163.45,64.4 163.45,60.97 163.79,60.63 | 163.83,64.78 123.19,64.78 | 123.19,64.78 74.93,64.78 | 74.93,64.78 60.71,64.78 38.73,64.78 | 38.73,64.78 33.34,64.78 23.5,64.78 15.24,64.78 1.91,64.78 | 41.27,102.88 4.45,102.88 4.45,96.53 4.45,71.13 4.45,63.51 161.93,63.51 161.93,61.61 162.56,60.97 5.71,60.97 1.91,64.78 | 41.27,102.88 50.16,102.88 50.8,102.88 69.85,102.88 77.47,102.88 | 77.47,102.88 125.73,102.88 | 125.73,102.88 160.02,102.88 161.93,104.79 161.93,106.69 | 163.22,64.44 163.83,64.78 | 163.83,64.78 163.83,69.84 U$14.TIP | X26.2 163.79,60.63 | 163.79,60.63 163.79,57.12 K2.1 158.88,51.96 161.93,48.91 161.93,24.27 K1.1 | K3.1 122.94,21.35 125.73,24.14 125.73,49.42 | 125.73,49.42 K4.1 | K5.1 74.55,21.22 77.47,24.14 77.47,49.16 K6.1 74.42,64.27 74.93,64.78 | K7.1 38.48,21.35 41.27,24.14 41.27,49.54 K8.1 38.61,64.66 38.73,64.78 | 125.73,49.42 125.73,49.54 123.19,52.08 123.19,64.78 | K12.1 125.73,151.14 125.73,125.74 | 125.73,125.74 125.73,125.62 K11.1 | K10.1 159.13,153.94 161.93,151.14 161.93,125.87 K9.1 159.13,122.82 161.93,120.03 161.93,107.33 | K14.1 74.68,153.94 77.47,151.14 77.47,125.87 K13.1 74.68,122.82 77.47,120.03 77.47,102.88 | K16.1 38.61,153.81 41.27,151.14 41.27,125.62 K15.1 41.27,120.03 41.27,102.88 | 161.93,107.33 161.93,106.69 | 125.73,125.74 123.19,123.2 123.19,122.57 125.73,120.03 125.73,102.88 | 8.26,104.79 23.5,104.79 | 159.38,104.79 160.02,104.79 161.93,106.69 | 23.5,104.79 159.38,104.79 | 159.38,104.79 161.93,107.33
N$4  (via drill 0.5)
  Top 0.254: IC1.15 v77.47,81.29 | RN1.3 114.45,96.04 115.57,97.17 115.57,98.44 116.2,99.07 118.75,99.07 JP1.A3
  Bottom 0.254: v77.47,81.29 75.56,81.29 74.93,81.93 74.93,99.07 76.2,100.34 119.38,100.34 120.02,99.71 JP1.A3
N$405  (via drill 0.5)
  Top 0.229: IC1.21 85.09,78.43 84.45,77.8 71.12,77.8 70.48,78.43 IC3.1
  Top 0.254: 85.09,78.43 v85.09,80.78 | v99.31,77.99 99.95,77.36 102.01,77.36
  Top 0.305: 102.01,77.36 102.07,77.36 RN19.5
  Bottom 0.229: v85.09,80.78 85.09,80.66 85.72,81.29 98.68,81.29 99.31,80.66 v99.31,77.99
N$406  (via drill 0.5)
  Top 0.229: IC1.25 v90.18,77.74 90.17,75.89 89.53,75.26 66.04,75.26 65.41,75.89 IC3.5 | v95.89,73.99 99.38,73.99 99.69,73.67 102,73.67 RN18.5
  Bottom 0.229: v90.18,77.74 90.17,78.9 90.53,79.26 95.48,79.26 95.89,78.86 v95.89,73.99
N$407  (via drill 0.5)
  Top 0.229: IC1.26 v91.44,77.74 91.44,75.58 90.49,74.62 64.77,74.62 64.14,75.26 IC3.6 | v96.84,73.04 99.38,73.04 99.69,72.72 101.99,72.72 RN18.6
  Bottom 0.229: v91.44,77.74 91.44,78.63 91.57,78.75 94.74,78.75 94.87,78.63 94.87,73.29 95.12,73.04 v96.84,73.04
N$408  (via drill 0.5)
  Top 0.254: IC1.16 v78.74,82.56 | RN1.2 114.94,95.24 115.57,95.9 116.2,96.53 118.75,96.53 JP1.A2
  Bottom 0.254: v78.74,82.56 76.2,82.56 75.56,83.2 75.56,98.44 76.83,99.71 118.11,99.71 118.75,99.07 118.75,96.53 JP1.A2
N$409  (via drill 0.5)
  Top 0.229: IC1.22 86.36,77.8 85.72,77.17 69.85,77.17 69.22,77.8 IC3.2
  Top 0.254: 86.36,77.8 v86.36,77.74 | v98.3,77.23 99.06,77.23 99.69,76.59 102.05,76.59 RN19.6
  Bottom 0.229: v86.36,77.74 86.36,80.4 86.74,80.78 97.79,80.78 98.3,80.28 v98.3,77.23
N$410  (via drill 0.5)
  Top 0.229: IC1.23 87.63,77.17 87,76.53 68.58,76.53 67.94,77.17 IC3.3
  Top 0.254: 87.63,77.17 v87.63,77.74 | v97.41,76.21 98.93,76.21 99.31,75.83 102.05,75.83 RN19.7
  Bottom 0.229: v87.63,77.74 87.63,80.02 87.88,80.28 97.03,80.28 97.41,79.9 v97.41,76.21
  Bottom 0.254: 97.66,76.09 v97.41,76.21
N$411  (via drill 0.5)
  Top 0.229: IC1.24 88.9,76.53 88.27,75.89 67.31,75.89 66.67,76.53 IC3.4
  Top 0.254: 88.9,76.53 v88.9,77.74 | v97.03,74.94 102,74.94 RN19.8
  Bottom 0.229: v88.9,77.74 88.9,79.26 89.41,79.77 95.76,79.77 96.52,79.01 96.52,75.45 v97.03,74.94
N$416  (via drill 0.6)
  Top 0.203: 69.22,87.01 69.53,87.32 75.25,87.32 76.2,88.28 76.2,90.5 76.83,91.14 93.34,91.14 93.98,91.77 v93.98,96.53
  Top 0.229: v93.98,96.53 93.98,97.42 93.22,98.18 93.22,98.96 RN21.8
  Top 0.406: v93.98,90.18 IC1.1 | IC4.8 69.22,87.01
  Bottom 0.406: v93.98,96.53 v93.98,90.18
N$417  (via drill 0.6)
  Top 0.203: IC4.7 67.94,87.32 68.45,87.83 74.74,87.83 75.56,88.66 75.56,91.14 76.2,91.77 92.08,91.77 92.71,92.4 v92.71,96.53
  Top 0.229: v92.71,96.53 92.71,97.55 92.33,97.93 92.33,99.02 RN21.7
  Top 0.406: v92.71,90.18 IC1.2
  Bottom 0.406: v92.71,96.53 v92.71,90.18
N$418  (via drill 0.6)
  Top 0.203: IC4.6 66.67,87.64 67.37,88.34 73.98,88.34 74.93,89.29 74.93,91.77 75.56,92.4 90.81,92.4 91.44,93.04 v91.44,96.53
  Top 0.229: v91.44,96.53 91.44,98.06 91.57,98.18 91.57,99.02 RN21.6
  Top 0.406: v91.44,90.18 IC1.3
  Bottom 0.406: v91.44,96.53 v91.44,90.18
N$419  (via drill 0.6)
  Top 0.203: IC4.5 65.41,87.64 66.61,88.85 73.34,88.85 74.3,89.8 74.3,92.4 74.93,93.04 89.53,93.04 90.17,93.67 v90.17,96.53
  Top 0.229: v90.17,96.53 90.17,97.68 90.68,98.18 90.68,98.96 RN21.5
  Top 0.406: v90.17,90.18 IC1.4
  Bottom 0.406: v90.17,90.18 v90.17,96.53
N$420  (via drill 0.6)
  Top 0.203: IC4.4 64.14,87.64 65.85,89.36 72.83,89.36 73.66,90.18 73.66,93.04 74.3,93.67 88.27,93.67 88.9,94.31 v88.9,96.53
  Top 0.229: v88.9,96.53 88.9,97.29 88.27,97.93 88.27,98.96 RN20.8
  Top 0.406: v88.9,90.18 IC1.5
  Bottom 0.406: v88.9,96.53 v88.9,90.18
N$421  (via drill 0.6)
  Top 0.203: IC4.3 62.87,87.64 65.09,89.87 72.33,89.87 73.03,90.56 73.03,93.67 73.66,94.31 87,94.31 87.63,94.95 v87.63,96.53
  Top 0.229: v87.63,96.53 87.63,97.68 87.38,97.93 87.38,99.02 RN20.7
  Top 0.406: v87.63,90.18 IC1.6
  Bottom 0.406: v87.63,96.53 v87.63,90.18
N$422  (via drill 0.6)
  Top 0.203: IC4.2 61.59,87.64 64.33,90.37 71.69,90.37 72.39,91.07 72.39,94.31 73.03,94.95 85.91,94.95 86.36,95.39 v86.36,96.53
  Top 0.229: IC1.7 86.36,88.28 | v86.36,96.53 86.36,97.55 86.61,97.8 86.61,99.02 RN20.6
  Top 0.406: 86.36,96.16 v86.36,96.53 | v86.36,90.18 IC1.7
  Bottom 0.406: v86.36,96.53 v86.36,90.18
N$423  (via drill 0.6)
  Top 0.203: IC4.1 60.33,87.64 63.69,91.01 71.18,91.01 71.75,91.58 71.75,94.87 72.47,95.58 84.64,95.58 85.09,96.03 v85.09,96.53
  Top 0.229: v85.09,96.53 85.09,97.55 85.72,98.18 85.72,98.96 RN20.5
  Top 0.406: v85.09,90.18 IC1.8
  Bottom 0.406: v85.09,90.18 v85.09,96.53
N$441
  Top 0.406: RN5.1 40.71,91.38 40.01,92.09 13.86,92.09 R16.C
N$442
  Top 0.406: RN8.7 RN7.2
N$443
  Top 0.406: RN7.3 RN8.6
N$444
  Top 0.406: RN8.5 RN7.4
N$445
  Top 0.406: RN5.2 40.24,90.58 39.37,91.45 17.03,91.45 R15.C
N$447
  Top 0.406: RN5.4 39.3,88.98 38.1,90.18 23.38,90.18 R13.C
N$448
  Top 0.406: RN5.5 RN6.4
N$449
  Top 0.406: RN7.1 RN8.8
N$450
  Top 0.406: RN8.1 39.44,87.57 37.47,89.55 26.55,89.55 R12.C
N$451
  Top 0.406: RN5.6 RN6.3
N$452
  Top 0.406: RN8.2 38.97,86.77 36.83,88.91 29.73,88.91 R11.C
N$453
  Top 0.406: RN6.2 RN5.7
N$454
  Top 0.406: RN5.8 RN6.1
N$458
  Top 0.406: RN5.3 39.77,89.78 38.73,90.82 20.2,90.82 R14.C
N$459
  Top 0.406: RN8.3 38.5,85.97 36.2,88.28 32.91,88.28 R10.C
N$463
  Top 0.406: RN12.4 RN11.5
N$470
  Top 0.406: RN8.4 38.03,85.17 36.2,87.01 35.67,87.01 R9.C
N$473
  Top 0.406: RN12.5 38.03,82.49 36.2,80.66 35.67,80.66 R1.C
N$474
  Top 0.406: RN11.6 RN12.3
N$475
  Top 0.406: RN12.6 38.5,81.69 36.2,79.39 32.91,79.39 R2.C
N$476
  Top 0.406: RN12.7 38.97,80.89 36.83,78.75 29.73,78.75 R3.C
N$477
  Top 0.406: RN9.4 RN10.5
N$478
  Top 0.406: RN10.6 RN9.3
N$479
  Top 0.406: RN9.2 RN10.7
N$480
  Top 0.406: RN10.8 RN9.1
N$481
  Top 0.406: RN12.2 RN11.7
N$482
  Top 0.406: RN10.1 39.3,78.68 38.1,77.48 23.38,77.48 R5.C
N$483
  Top 0.406: RN12.8 39.44,80.09 37.47,78.12 26.55,78.12 R4.C
N$484
  Top 0.406: RN10.3 40.24,77.08 39.37,76.21 17.03,76.21 R7.C
N$485
  Top 0.406: RN10.4 40.71,76.28 40.01,75.58 13.86,75.58 R8.C
N$486
  Top 0.406: RN10.2 39.77,77.88 38.73,76.85 20.2,76.85 R6.C
N$498  (via drill 0.5)
  Top 0.254: IC1.17 80.01,83.2 v79.38,83.83 | RN1.1 115.75,94.44 116.2,93.99 118.75,93.99 JP1.A1
  Bottom 0.254: v79.38,83.83 76.83,83.83 76.2,84.47 76.2,97.8 77.47,99.07 115.57,99.07 116.2,98.44 116.2,92.09 116.84,91.45 118.75,91.45 JP1.A1
N$500
  Top 0.406: RN11.8 RN12.1
N$513
  Top 0.813: CB1.2 CA1.2 139.29,70.27 138.43,71.13 IC7.8
  Top 1.27: BRA1.+ 157.16,70.63 156.71,70.18 143.91,70.18 CB1.2
N$515
  Top 0.254: POWER.A 149.75,82.04 148.27,83.51 146.3,83.51 RNB.3
  Top 0.305: RNB.3 146.15,83.64
N$516
  Top 0.254: RNB.4 147,84.46 148.27,85.74 150.38,85.74 I2C.A
  Top 0.305: RNB.4
N$517  (via drill 0.6)
  Top 0.254: RNE.5 165.2,89.39 v165.23,89.42
  Bottom 0.254: v165.23,89.42 160.15,89.42 160.02,89.55 138.43,89.55 137.16,90.82 137.16,97.48 136.84,97.8 U$16.A1
N$518  (via drill 0.6)
  Top 0.254: RNE.6 162.32,89 161.93,88.59 v159.51,88.59
  Bottom 0.254: U$16.B1 135.25,95.26 135.89,94.63 135.89,89.55 137.16,88.28 159.19,88.28 v159.51,88.59
N$524
  Bottom 2.54: 164.47,69.86 163.83,69.86
N$525  (via drill 0.5)
  Top 0.229: IC3.7 62.87,74.62 63.5,73.99 91.76,73.99 92.71,74.94 v92.71,77.74 IC1.27 | v97.79,72.09 101.52,72.09 RN18.7
  Bottom 0.229: v97.79,72.09 93.03,72.09 92.71,72.4 v92.71,77.74
N$526
  Top 0.229: IC1.28 93.98,73.99 | 93.98,73.99 93.34,73.36 62.23,73.36 61.59,73.99 IC3.8 | 93.98,73.99 93.98,71.77 94.61,71.13 102,71.13 RN18.8
OC_R1_A  (via drill 0.6)
  Top 0.406: IC3.18 v70.48,69.93 71.82,68.59 149.86,68.59 151.76,66.69 151.76,59.7 154.94,56.53 159.38,56.53 161.29,54.62 161.29,13.47 K1.2 | RN11.4 58.35,82.49 v58.55,82.31
  Bottom 0.406: v58.55,82.31 70.1,82.31 70.48,81.93 v70.48,69.93
OC_R1_B
  Top 0.203: RN7.5 57.22,85.17 63.82,91.77 68.26,91.77 69.22,92.72 IC4.11
  Top 0.406: IC4.11 69.22,100.34 69.85,100.98 80.64,100.98 81.28,101.61 128.91,101.61 130.18,102.88 157.48,102.88 158.75,104.15 158.75,112.53 K9.2
OC_R2_A  (via drill 0.6)
  Top 0.406: RN11.3 56.75,81.69 v57.15,81.29 | IC3.17 v69.22,69.93 69.26,67.99 69.94,67.32 147.96,67.32 150.5,64.78 150.5,59.07 156.84,52.72 156.84,43.83 158.62,42.05 K2.2
  Bottom 0.406: v57.15,81.29 67.94,81.29 69.22,80.02 v69.22,69.93
OC_R2_B
  Top 0.203: IC4.12 67.94,93.36 66.99,92.4 63.82,92.4 57.38,85.97 RN7.6
  Top 0.406: IC4.12 67.94,100.98 68.58,101.61 80.01,101.61 80.64,102.25 128.27,102.25 129.54,103.52 156.21,103.52 156.84,104.15 156.84,141.74 K10.2
OC_R3_A  (via drill 0.6)
  Top 0.406: RN11.2 55.01,80.89 v55.88,80.02 | IC3.16 v67.94,69.93 67.94,66.69 68.58,66.05 124.46,66.05 125.73,64.78 125.73,13.98 122.94,11.19 K3.2
  Bottom 0.406: v55.88,80.02 66.67,80.02 67.94,78.75 v67.94,69.93
OC_R3_B
  Top 0.203: RN7.7 57.55,86.77 63.82,93.04 66.36,93.04 66.67,93.36 IC4.13
  Top 0.406: IC4.13 66.67,101.61 67.31,102.25 79.38,102.25 80.01,102.88 121.92,102.88 122.56,103.52 122.56,112.28 K11.2
OC_R4_A  (via drill 0.6)
  Top 0.406: RN11.1 53.27,80.09 v54.61,78.75 | IC3.15 v66.67,69.93 66.67,66.05 67.94,64.78 119.38,64.78 120.65,63.51 120.65,44.46 122.94,42.18 K4.2
  Bottom 0.406: v54.61,78.75 65.41,78.75 66.67,77.48 v66.67,69.93
OC_R4_B
  Top 0.203: RN7.8 57.72,87.57 63.82,93.67 65.09,93.67 65.41,93.99 IC4.14
  Top 0.406: IC4.14 65.41,102.25 66.04,102.88 78.74,102.88 79.44,103.58 120.02,103.58 120.9,104.47 120.9,141.74 K12.2
OC_R5_A  (via drill 0.6)
  Top 0.406: RN9.8 52.14,78.68 53.34,77.48 v58.42,77.48 | IC3.14 v65.41,69.93 65.41,65.73 77.47,53.67 77.47,14.11 K5.2
  Bottom 0.406: v58.42,77.48 64.14,77.48 65.41,76.21 v65.41,69.93
OC_R5_B
  Top 0.203: IC4.15 64.14,94.63 63.82,94.31 63.5,94.31 58.17,88.98 RN6.5
  Top 0.406: IC4.15 64.14,102.88 64.77,103.52 73.03,103.52 74.55,105.04 74.55,112.53 K13.2
OC_R6_A  (via drill 0.6)
  Top 0.406: RN9.7 51.67,77.88 53.34,76.21 v57.15,76.21 | IC3.13 v64.14,69.93 64.14,65.42 72.39,57.16 72.39,44.08 K6.2
  Bottom 0.406: v57.15,76.21 62.87,76.21 64.14,74.94 v64.14,69.93
OC_R6_B
  Top 0.203: RN6.6 58.02,89.78 62.87,94.63 IC4.16
  Top 0.406: IC4.16 62.87,103.52 64.14,104.79 70.48,104.79 72.39,106.69 72.39,141.74 K14.2
OC_R7_A  (via drill 0.6)
  Top 0.406: RN9.6 51.2,77.08 53.34,74.94 v55.88,74.94 | IC3.12 v62.87,69.93 62.87,67.32 62.23,66.69 42.55,66.69 41.27,65.42 41.27,13.35 38.99,11.06 K7.2
  Bottom 0.406: v55.88,74.94 61.59,74.94 62.87,73.67 v62.87,69.93
OC_R7_B
  Top 0.203: RN6.7 57.87,90.58 61.59,94.31 IC4.17
  Top 0.406: IC4.17 61.59,101.61 60.96,102.25 38.73,102.25 38.35,102.63 38.35,112.53 K15.2
OC_R8_A  (via drill 0.6)
  Top 0.406: RN9.5 50.73,76.28 53.34,73.67 v54.61,73.67 | IC3.11 v61.59,69.93 61.59,68.59 60.96,67.96 36.83,67.96 35.56,66.69 35.56,45.1 K8.2
  Bottom 0.406: v54.61,73.67 60.33,73.67 61.59,72.4 v61.59,69.93
OC_R8_B
  Top 0.203: RN6.8 57.72,91.38 60.33,93.99 IC4.18
  Top 0.406: IC4.18 60.33,100.98 59.69,101.61 37.15,101.61 36.45,102.31 36.45,141.62 K16.2
REG_5V  (via drill 0.6)
  Top 0.254: RNB.6 143.97,83.66 143.51,83.2 143.51,80.34 143.83,80.02 CB2.2 | 137.03,79.51 130.05,79.51 129.54,80.02 | 101.69,87.09 101.69,89 103.25,90.56 107.77,90.56 RN17.2 RN17.1 107.95,91.55 107.95,92.72 108.58,93.36 112.39,93.36 113.03,92.72 JP1.B1
  Top 0.305: 81.28,85.1 82.55,86.37 83.19,86.37 83.82,87.01 | IC1.18 v81.28,84.47 | IC1.9 83.82,87.01 | 83.82,87.01 84.45,86.37 94.93,86.37 95.25,86.37
  Top 0.813: CB2.2 CA2.2 139.29,78.35 138.43,77.48 | 138.43,77.48 IC7.1 | 137.03,79.51 137.67,79.51 138.43,78.75 138.43,77.48
  Top 1.016: CB2.2 144.06,78.12 147.32,78.12 147.96,77.48 C27.+ | 129.54,80.02 125.73,80.02 124.46,78.75 C26.+ 114.3,74.31 112.39,76.21 107.95,76.21 107.31,75.58 | 107.31,75.58 107.31,77.74 106.55,78.5 102.49,78.5 101.69,79.3 C1.1 C4.1 101.69,86.92 | 107.31,75.58 C25.+ | C6.1 96.29,85.33 95.25,86.37 | C6.1 C7.1 | 101.69,86.92 100.97,87.64 97.16,87.64 96.52,87.01 96.52,85.33 C6.1 | 101.69,86.92 101.69,87.09
  Top 1.27: 137.16,79.39 130.18,79.39 129.54,80.02 129.54,94.95 U$16.B2 | 94.93,86.37 84.14,86.37 83.82,86.69 82.87,86.69 81.28,85.1 v81.28,84.47
  Bottom 0.254: JP1.B3 JP1.B2 JP1.B1
  Bottom 0.813: U$16.B2 U$16.A2
  Bottom 1.27: C24.+ v81.28,84.47
REG_5V_BUS
  Top 0.254: 165.99,80.34 159.07,80.34 158.75,80.66 158.75,86.37 158.43,86.69 145.41,86.69 144.78,86.06 144.78,84.46 RNB.5
  Top 0.61: X25.3 165.99,80.34 | X27.2 166.12,97.1
  Bottom 0.406: 165.99,80.34 X25.3 | 166.12,97.1 X27.2
  Bottom 0.813: 165.99,80.34 167.64,80.34 168.91,81.61 168.91,95.83 167.64,97.1 166.12,97.1

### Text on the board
tNames: Bank 2 | 8 | 6 | 4 | 2 | 7 | 5 | 3 | 1 | MCP23017 | I2CR16x0 | REV.A | I2C 5V | Address: | PULL-UP | GND | +5V | A0 | 2016 ControlEverything.com | A1 | SDA | SCL | A2 | I2C OUT | SCL | SDA | +5V | I2C IN | GND | 12V DC / Power / Supply | 8 | 6 | 4 | 2 | 7 | 5 | 3 | 1 | Bank 1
